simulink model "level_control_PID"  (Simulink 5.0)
settings: Solver=ode45  StartTime=0.0  StopTime=50  RelTol=1e-6
libraries: simulink x1

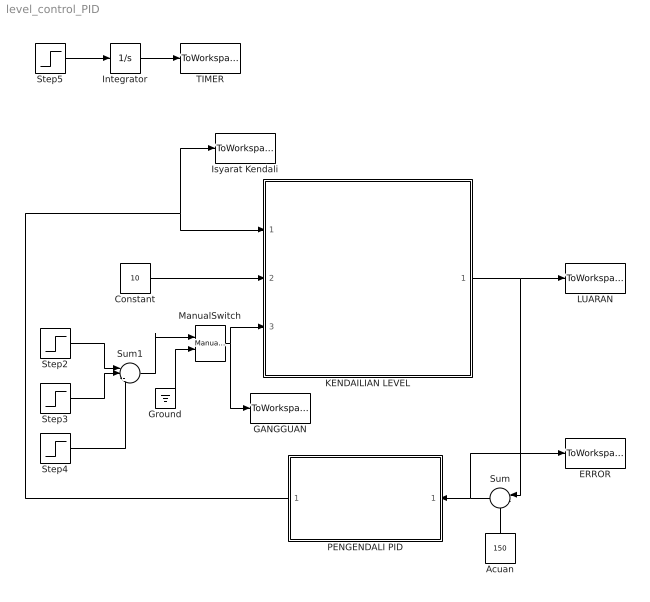
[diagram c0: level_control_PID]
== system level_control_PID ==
  Acuan : Constant  Orientation=up  Value=150
  Constant : Constant  Value=10
  ERROR : ToWorkspace  VariableName=error  SampleTime=-1  SaveFormat=Array
  GANGGUAN : ToWorkspace  VariableName=gangguan  SampleTime=-1  SaveFormat=Array
  Ground : Ground
  Integrator : Integrator
  Isyarat Kendali : ToWorkspace  VariableName=pompa  SampleTime=-1  SaveFormat=Array
  KENDAILIAN LEVEL : Subsystem
  LUARAN : ToWorkspace  VariableName=level  SampleTime=-1  SaveFormat=Array
  ManualSwitch : simulink/Signal Routing/Manual Switch  sw=1  action=0
  PENGENDALI PID : Subsystem  Orientation=left
  Step2 : Step  Time=9  After=10  SampleTime=0
  Step3 : Step  Time=12  SampleTime=0
  Step4 : Step  Time=14  SampleTime=0
  Step5 : Step  Time=0  SampleTime=0
  Sum : Sum  Orientation=left  Inputs=|-+
  Sum1 : Sum  Inputs=|+--
  TIMER : ToWorkspace  VariableName=time  SampleTime=-1  SaveFormat=Array
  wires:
  Constant/1 -> KENDAILIAN LEVEL/2(KATUP manual)
  Step2/1 -> Sum1/1
  Step3/1 -> Sum1/2
  Step4/1 -> Sum1/3
  KENDAILIAN LEVEL/1(level) -> LUARAN/1, Sum/1
  Step5/1 -> Integrator/1
  Integrator/1 -> TIMER/1
  ManualSwitch/1 -> KENDAILIAN LEVEL/3(KATUP otomatis), GANGGUAN/1
  Sum1/1 -> ManualSwitch/1
  Ground/1 -> ManualSwitch/2
  Sum/1 -> PENGENDALI PID/1(error), ERROR/1
  Acuan/1 -> Sum/2
  PENGENDALI PID/1(kecepatan pompa) -> KENDAILIAN LEVEL/1(pengendali POMPA), Isyarat Kendali/1

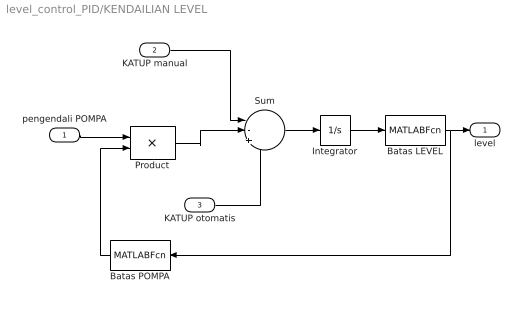
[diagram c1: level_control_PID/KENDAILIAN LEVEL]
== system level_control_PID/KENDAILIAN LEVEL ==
  pengendali POMPA : Inport
  KATUP manual : Inport  Port=2
  KATUP otomatis : Inport  Port=3
  Batas LEVEL : MATLABFcn  MATLABFcn=batas_level
  Batas POMPA : MATLABFcn  Orientation=left  MATLABFcn=batas_pompa
  Integrator : Integrator  InitialCondition=200
  Product : Product
  Sum : Sum  Inputs=|-+-
  level : Outport
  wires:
  Batas LEVEL/1 -> level/1, Batas POMPA/1
  Integrator/1 -> Batas LEVEL/1
  Sum/1 -> Integrator/1
  KATUP manual/1 -> Sum/1
  KATUP otomatis/1 -> Sum/3
  pengendali POMPA/1 -> Product/1
  Batas POMPA/1 -> Product/2
  Product/1 -> Sum/2

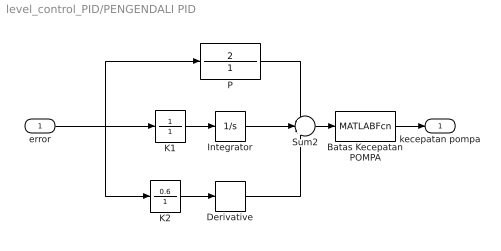
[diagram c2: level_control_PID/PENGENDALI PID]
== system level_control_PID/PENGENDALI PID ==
  error : Inport
  Batas Kecepatan POMPA : MATLABFcn  MATLABFcn=batas_kec_pompa
  Derivative : Derivative
  Integrator : Integrator
  K1 : TransferFcn  Numerator=1  Denominator=1
  K2 : TransferFcn  Numerator=0.6  Denominator=1
  P : TransferFcn  Numerator=2  Denominator=1
  Sum2 : Sum  Inputs=+++
  kecepatan pompa : Outport
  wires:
  Batas Kecepatan POMPA/1 -> kecepatan pompa/1
  K1/1 -> Integrator/1
  K2/1 -> Derivative/1
  Sum2/1 -> Batas Kecepatan POMPA/1
  Integrator/1 -> Sum2/2
  P/1 -> Sum2/1
  error/1 -> K1/1, P/1, K2/1
  Derivative/1 -> Sum2/3
